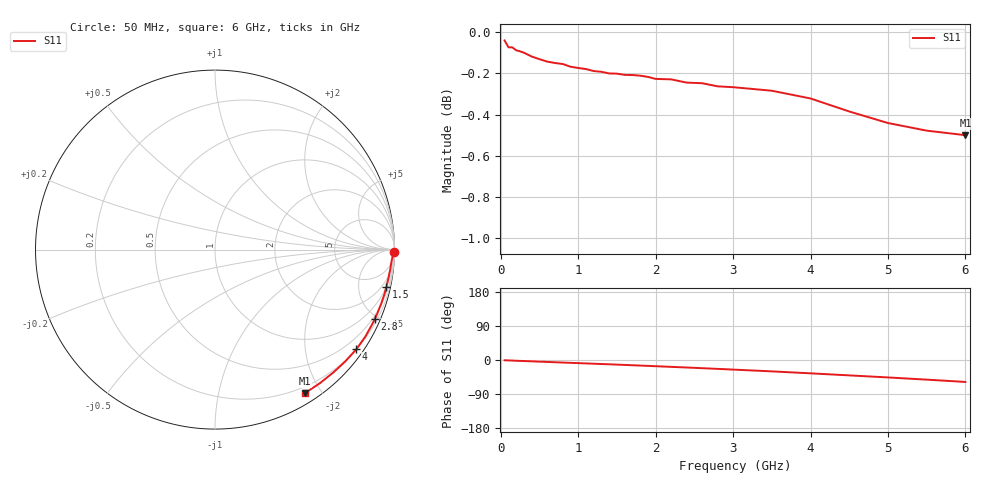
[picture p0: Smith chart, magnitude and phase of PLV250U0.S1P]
! Infineon Technologies  Discrete & RF Semiconductors
! BAR 64-04W /-05W /-06W
! Si PIN Diode in SOT323
! VR = 0.25 V
! S-Parameters:  October  2008
# GHz  S  MA  R  50
!  f  S11
! GHz  MAG  ANG
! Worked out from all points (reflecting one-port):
!   34 points, 50 MHz to 6 GHz, reference 50 ohm
!   lowest |S11| = -0.5 dB at 6 GHz (marker M1), VSWR 34.74, Z = 6.13 - j90.1 ohm
!   phase of S11 starts at -1 deg and turns -57 deg over the sweep
!   S11 on the Smith chart (normalised r, x): 50 MHz: open; 1.5 GHz: 1.01, -9.25; 2.8 GHz: 0.37, -4.80; 4 GHz: 0.20, -3.14; 6 GHz: 0.12, -1.80
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0.05  0.9954 -0.7
0.1  0.9916 -1.1
0.15  0.9916 -1.5
0.2  0.99 -2.0
0.25  0.9894 -2.4
0.3  0.9886 -2.7
0.4  0.9865 -3.5
0.5  0.9851 -4.4
0.6  0.9837 -5.1
0.8  0.9824 -6.7
0.9  0.9809 -7.5
1  0.9802 -8.2
1.3  0.9781 -10.6
1.4  0.9772 -11.3
1.5  0.9771 -12.2
1.6  0.9765 -13.0
1.9  0.9754 -15.5
2.2  0.974 -18.1
2.4  0.9722 -19.8
2.6  0.9719 -21.6
2.8  0.9702 -23.4
3  0.9697 -25.3
3.5  0.9678 -30.0
4  0.9636 -35.2
4.5  0.9567 -40.6
5  0.9505 -46.0
5.5  0.9465 -51.8
6  0.944 -57.9
